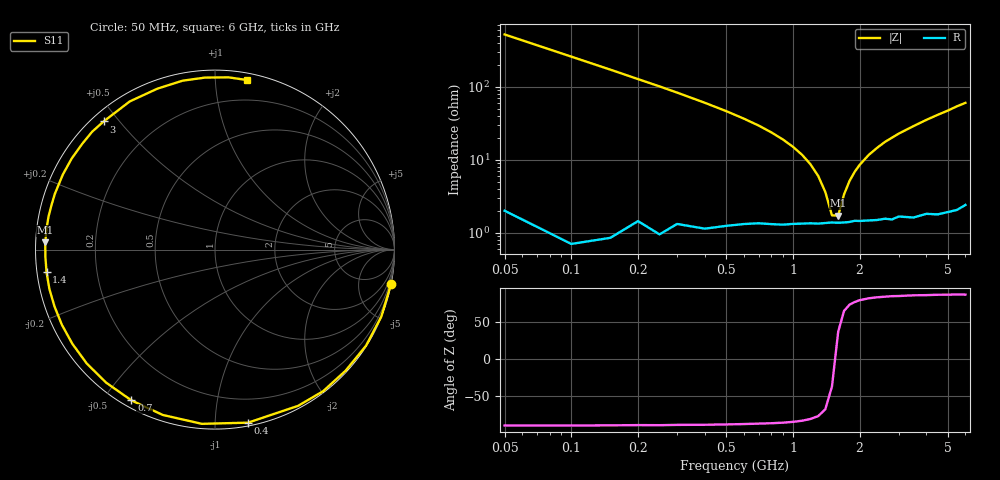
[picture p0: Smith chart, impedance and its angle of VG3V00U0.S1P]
! Infineon Technologies  Discrete & RF Semiconductors
! BB 831
! Si Tuning Diode in SOD323
! VR = 3 V
! S-Parameters:  July  1999
# GHz  S  MA  R  50
!  f  S11
! GHz  MAG  ANG
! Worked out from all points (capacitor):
!   34 points, 50 MHz to 6 GHz, reference 50 ohm
!   read as one part to ground: C = 6.13 pF near 50 MHz
!   lowest |Z| = 1.73 ohm at 1.6 GHz (marker M1)
!   series resonance near 1.55 GHz, so ESL is about 1.7 nH
!   S11 on the Smith chart (normalised r, x): 50 MHz: 0, -10; 400 MHz: 0.02, -1.21; 700 MHz: 0.03, -0.59; 1.4 GHz: 0.03, -0.07; 3 GHz: 0.03, +0.46; 6 GHz: 0.05, +1.20
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0.05  0.9993 -11.0
0.1  0.999 -21.9
0.15  0.9973 -32.5
0.2  0.9923 -42.9
0.25  0.9925 -52.6
0.3  0.986 -62.0
0.4  0.9816 -79.2
0.5  0.9735 -94.3
0.6  0.9662 -107.5
0.7  0.9605 -119.0
0.8  0.9578 -129.3
0.9  0.9556 -138.4
1  0.9524 -146.5
1.1  0.9504 -153.8
1.2  0.9487 -160.5
1.4  0.947 -172.3
1.6  0.9465 177.6
1.8  0.9456 168.7
2  0.9449 160.9
2.4  0.9461 147.5
2.6  0.9458 141.4
3  0.946 131.0
3.5  0.9524 119.9
4  0.9523 109.7
4.5  0.9582 100.9
5  0.96 93.3
5.5  0.9626 85.5
6  0.9614 79.4
